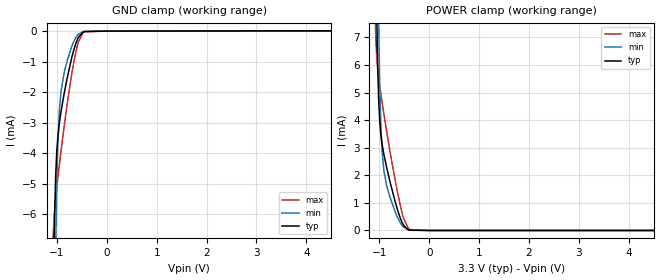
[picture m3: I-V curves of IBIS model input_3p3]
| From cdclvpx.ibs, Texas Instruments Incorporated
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|   Input_3p3 Model   |
[Model]   input_3p3
Model_type   Input
| Signals   INN0, INP0, INN1, INP1
| variable   typ   min   max
C_comp   0.295pF   0.292pF   0.298pF
Vinl = 0.85V   |
Vinh = 2.40V   |
| Where nom  PVT is Nominal Process, 3.3V, 40C
|   Fast PVT is Strong Process,  3.6V, -40C
|   Slow PVT is Weak Process,   2.375V,100C
[Model Spec]
|   VCC=3.3V   VCC=2.375V   VCC=3.6V
Vinl   0.85V   0.00V   1.70V
Vinh   2.40V   1.20V   3.60V
| Junction Temperature (Ambient temp is 25C typ, 85C min, -40C max)
[Temperature Range]   40C   100C   -40C
[Voltage range]   3.3V   2.375V   3.6V
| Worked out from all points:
|   GND clamp passes 1 mA (typ) near -0.72 V on its own axis
|   POWER clamp passes 1 mA (typ) near -0.68 V on its own axis
[GND Clamp]
|   Voltage   I(typ)   I(min)   I(max)
-3.3V     -1.065A    -1.072A    -1.061A
-1.08V    -10.1mA    -17.36mA   -6.92mA
-1.062V   -7.721mA   -13.48mA   -6.284mA
-1.045V   -6.08mA    -10.32mA   -5.865mA
-1.02V    -4.586mA   -6.821mA   -5.406mA
-981mV    -3.472mA   -3.738mA   -4.815mA
-953.3mV  -3.048mA   -2.69mA    -4.426mA
-916.6mV  -2.634mA   -1.973mA   -3.929mA
-842mV    -1.944mA   -1.279mA   -2.969mA
-673.6mV  -692.5uA   -387.6uA   -1.133mA
-476.1mV  -32.92uA   -17.23uA   -49.69uA
6.598V    12.89uA    10.05uA    17.3uA
[POWER Clamp]
|   Voltage   I(typ)   I(min)   I(max)
-3.3V     1.072A     1.078A     1.069A
-1.079V   11.93mA    20.27mA    7.424mA
-1.05V    7.485mA    13.33mA    6.212mA
-1.013V   4.696mA    7.33mA     5.512mA
-988mV    3.851mA    4.944mA    5.176mA
-965.6mV  3.405mA    3.623mA    4.895mA
-943.5mV  3.104mA    2.832mA    4.627mA
-909.2mV  2.752mA    2.158mA    4.223mA
-780mV    1.716mA    1.167mA    2.788mA
-631.5mV  723uA      453.1uA    1.342mA
-426.6mV  37.46uA    23.34uA    99.56uA
6.598V    0A         0A         0A
